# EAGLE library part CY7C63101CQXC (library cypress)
Universal Serial Bus Microcontroller Integrated USB transceiver Source: www.cypress.com .. CY7C6301XX.pdf
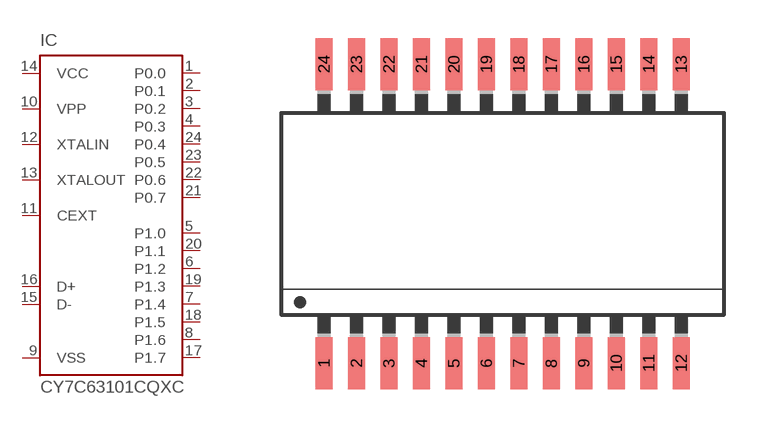
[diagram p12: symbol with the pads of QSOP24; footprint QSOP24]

Designator prefix IC

## CY7C63101CQXC (MPN: CY7C63101C-QXC; OC_FARNELL: unknown; OC_NEWARK: 19M7035)  [QSOP24]
1  P0.0
2  P0.1
3  P0.2
4  P0.3
5  P1.0
6  P1.2
7  P1.4
8  P1.6
9  VSS  pwr
10  VPP  in
11  CEXT  pas
12  XTALIN  in
13  XTALOUT  out
14  VCC  pwr
15  D-
16  D+
17  P1.7
18  P1.5
19  P1.3
20  P1.1
21  P0.7
22  P0.6
23  P0.5
24  P0.4

## Footprint QSOP24 (pad centres in mm)
24-Lead Quarter Size Outline Q13 Source: www.cypress.com .. CY7C6301XX.pdf
smd 0.66 x 2.032: 1 -6.985,-5.842; 2 -5.715,-5.842; 3 -4.445,-5.842; 4 -3.175,-5.842; 5 -1.905,-5.842; 6 -0.635,-5.842; 7 0.635,-5.842; 8 1.905,-5.842; 9 3.175,-5.842; 10 4.445,-5.842; 11 5.715,-5.842; 12 6.985,-5.842; 13 6.985,5.842; 14 5.715,5.842; 15 4.445,5.842; 16 3.175,5.842; 17 1.905,5.842; 18 0.635,5.842; 19 -0.635,5.842; 20 -1.905,5.842; 21 -3.175,5.842; 22 -4.445,5.842; 23 -5.715,5.842; 24 -6.985,5.842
